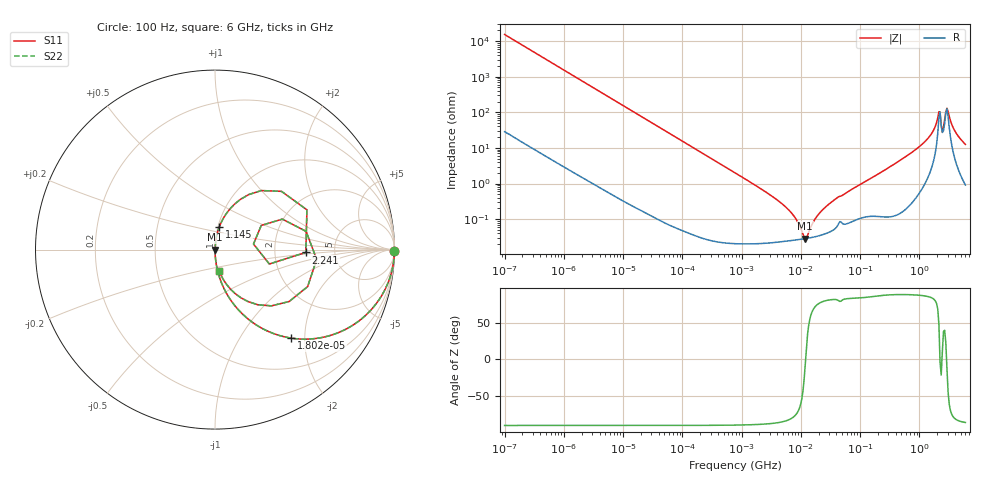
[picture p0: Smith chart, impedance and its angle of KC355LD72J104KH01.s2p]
!Murata Part Number: KC355LD72J104KH01
!These Parameters are Measured in Series Mode Connection
!Data Generated on Jun 19, 2026
!  o--ll--o
!Port1  Port2
!  o------o
!Operation Temp=25[degC], DC Bias Voltage=0[V]
!Freq. Start=100[Hz] Stop=6[GHz] 401[Steps]
# Hz S RI R 50
!Freq.(Hz) S11(Real) S11(Imag) S21(Real) S21(Imag) S12(Real) S12(Imag) S22(Real) S22(Imag)
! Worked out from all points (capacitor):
!   401 points, 100 Hz to 6 GHz, reference 50 ohm
!   read as one part in series: C = 103 nF near 109 Hz
!   lowest |Z| = 28.4 mohm at 11.89 MHz (marker M1)
!   series resonance near 12.04 MHz, so ESL is about 1.7 nH
!   S11 on the Smith chart (normalised r, x): 100 Hz: open; 18.02 kHz: 1.00, -1.72; 1.145 GHz: 1.02, +0.26; 2.241 GHz: 3.04, -0.13; 6 GHz: 1.02, -0.25
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100  0.9999 -0.00649  5.42e-05 0.00649  5.42e-05 0.00649  0.9999 -0.00649
2008  0.9832 -0.1277  0.0168 0.1277  0.0168 0.1277  0.9832 -0.1277
6433  0.8522 -0.3539  0.1478 0.3539  0.1478 0.3539  0.8522 -0.3539
18016  0.4255 -0.4933  0.5745 0.4933  0.5745 0.4933  0.4255 -0.4933
40335  0.1295 -0.3346  0.8705 0.3346  0.8705 0.3346  0.1295 -0.3346
141303  0.0123 -0.1086  0.9877 0.1086  0.9877 0.1086  0.0123 -0.1086
774597  0.000603 -0.02  0.9994 0.02  0.9994 0.02  0.000603 -0.02
5311619  0.000242 -0.00233  0.9998 0.00233  0.9998 0.00233  0.000242 -0.00233
7947587  0.000258 -0.00109  0.9997 0.00109  0.9997 0.00109  0.000258 -0.00109
1.189169e7  0.000282 -3.04e-05  0.9997 3.04e-05  0.9997 3.04e-05  0.000282 -3.04e-05
1.555665e7  0.000306 0.000656  0.9997 -0.000656  0.9997 -0.000656  0.000306 0.000656
2.225763e7  0.000358 0.00165  0.9996 -0.00165  0.9996 -0.00165  0.000358 0.00165
3.80911e7  0.000554 0.00357  0.9994 -0.00357  0.9994 -0.00357  0.000554 0.00357
3.124326e8  0.00197 0.0286  0.998 -0.0286  0.998 -0.0286  0.00197 0.0286
1.144649e9  0.0242 0.1273  0.9758 -0.1273  0.9758 -0.1273  0.0242 0.1273
1.873145e9  0.187 0.3063  0.813 -0.3063  0.813 -0.3063  0.187 0.3063
2.048624e9  0.3705 0.3246  0.6295 -0.3246  0.6295 -0.3246  0.3705 0.3246
2.240541e9  0.506 -0.0156  0.494 0.0156  0.494 0.0156  0.506 -0.0156
2.679998e9  0.3753 0.1698  0.6247 -0.1698  0.6247 -0.1698  0.3753 0.1698
3.065283e9  0.5162 -0.2061  0.4838 0.2061  0.4838 0.2061  0.5162 -0.2061
3.505958e9  0.2383 -0.3073  0.7617 0.3073  0.7617 0.3073  0.2383 -0.3073
6e9  0.0241 -0.1214  0.9759 0.1214  0.9759 0.1214  0.0241 -0.1214
